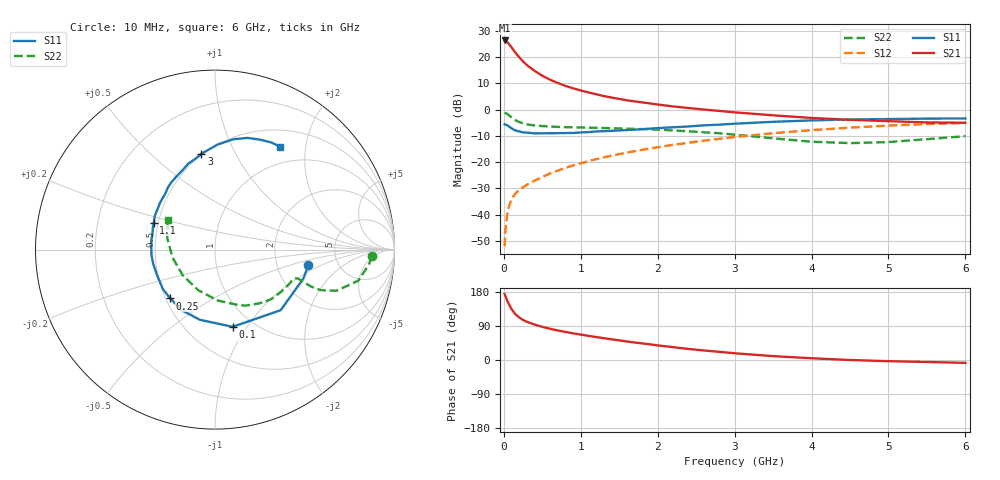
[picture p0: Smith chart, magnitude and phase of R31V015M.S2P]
! SIEMENS Small Signal Semiconductors
! BFR181
! Si NPN RF Bipolar Junction Transistor in SOT23
! VCE = 1 V  IC = 15 mA
! Common Emitter S-Parameters:  May  1996
# GHz  S  MA  R  50
!  f  S11  S21  S12  S22
! GHz  MAG  ANG  MAG  ANG  MAG  ANG  MAG  ANG
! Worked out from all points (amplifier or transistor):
!   36 points, 10 MHz to 6 GHz, reference 50 ohm
!   highest |S21| = 26.4 dB at 10 MHz (marker M1)
!   |S21| within 3 dB of that: start of sweep to 109.2 MHz
!   unconditionally stable (mu >= 1): start of sweep to 19.1 MHz; 216.9 MHz to end of sweep
!   at 250 MHz: K = 1.08, MAG = 22.2 dB, |S12| = -29.5 dB
!   at 1.4 GHz: K = 1.45, MAG = 7.1 dB, |S12| = -17.6 dB
!   at 6 GHz: K = 1.13, MAG = -2.1 dB, |S12| = -5.1 dB
!   S11 on the Smith chart (normalised r, x): 10 MHz: 3.04, -0.72; 100 MHz: 0.81, -0.86; 250 MHz: 0.53, -0.33; 1.1 GHz: 0.47, +0.17; 3 GHz: 0.49, +0.74; 6 GHz: 0.73, +1.56
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0.01  0.5275 -9.3  20.81 174.4  0.0025 82.5  0.8743 -2.5
0.02  0.5185 -18.1  20.52 168.7  0.005 77.2  0.8631 -5.3
0.05  0.4978 -42.7  19.04 153.8  0.012 72.1  0.8176 -12.2
0.1  0.4413 -77.1  15.37 134.4  0.0198 64.4  0.7149 -18.7
0.15  0.4001 -102.2  12.2 120.7  0.0253 60.0  0.6309 -21.0
0.2  0.3852 -119.0  9.975 112.2  0.0294 59.9  0.5807 -21.1
0.25  0.3689 -132.5  8.27 105.6  0.0334 59.2  0.5487 -20.6
0.3  0.3642 -142.8  7.05 100.7  0.037 61.1  0.5248 -20.1
0.4  0.3526 -156.9  5.474 93.6  0.0443 63.7  0.4992 -19.4
0.5  0.3534 -167.4  4.431 87.5  0.0521 66.0  0.486 -19.3
0.6  0.3553 -175.4  3.725 82.5  0.0608 67.4  0.4761 -19.7
0.7  0.3557 176.7  3.223 78.0  0.0687 68.5  0.4686 -20.6
0.8  0.3586 170.9  2.835 74.1  0.0777 68.8  0.4642 -21.5
1.1  0.3729 156.2  2.125 63.8  0.1045 69.7  0.4539 -25.5
1.3  0.3885 147.4  1.814 57.5  0.1232 69.2  0.4467 -28.5
1.6  0.4081 136.1  1.505 48.8  0.1518 67.9  0.4337 -33.9
2.2  0.4608 117.8  1.15 33.8  0.2132 63.5  0.401 -46.3
3  0.5394 98.1  0.888 17.8  0.2999 54.9  0.3331 -67.7
3.5  0.586 88.5  0.779 10.2  0.3553 48.4  0.2842 -87.0
4.5  0.6481 73.8  0.64 0.0  0.4543 34.0  0.2301 -141.0
5.5  0.6741 62.4  0.57 -5.3  0.5301 19.2  0.2736 166.4
6  0.6789 57.7  0.563 -7.5  0.5574 11.8  0.312 147.6
